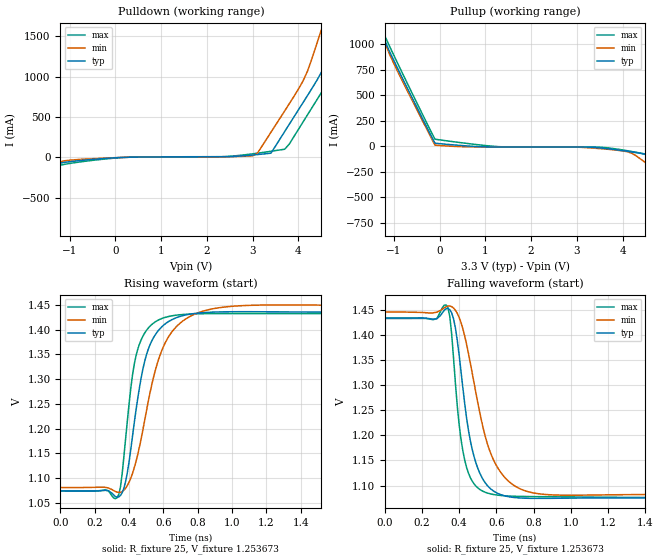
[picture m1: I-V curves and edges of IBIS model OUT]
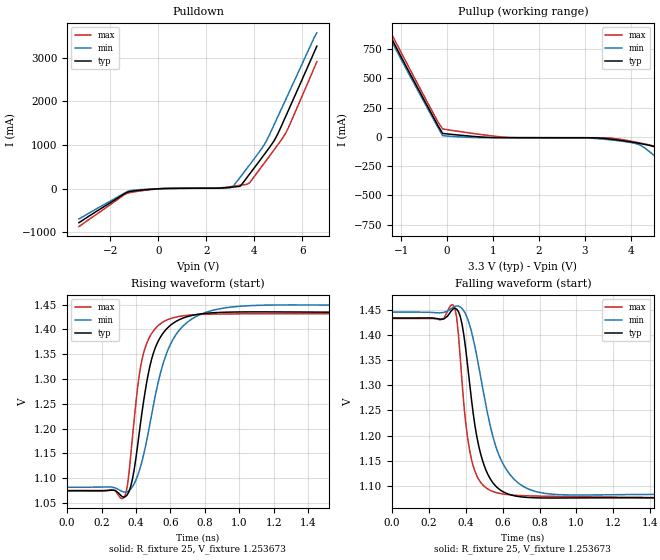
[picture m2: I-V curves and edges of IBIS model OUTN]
|   IBIS File of SG2520VHN C
|   LVDS, Vcc=3.3V, Io=7mA, fo<=212.5MHz
[IBIS Ver]   3.2
[File Name]   sg2520vhn_7m_33v.ibs
[File Rev]   1.0
[Date]   Sep. 23, 2020
[Source]
Fairchild Ensigna Lab's Method
[Notes]
Created by Minoru Kozaki
[Disclaimer]
Seiko Epson Corporation makes no warranty with respect to the
information contained herein.
[Copyright]
Copyright(C) 2020, Seiko Epson Corporation. All rights reserved.
|   Component
[Component]   SG2520VHN
[Manufacturer]  Seiko Epson Corporation
[Package]
R_pkg   17.7m   NA   NA
L_pkg   235p   NA   NA
C_pkg   208f   NA   NA
[Pin]   signal_name   model_name   R_pin   L_pin   C_pin
1   OE/ST   NC
2   NC   NC
3   GND   GND
4   OUT   OUT   17.7m   235p   208f
5   OUTN   OUTN   10.4m   129p   221f
6   VCC   POWER
[Diff Pin] inv_pin  vdiff  tdelay_typ
4   5   0   0
| Models and submodels in the file (2): OUT (Output), OUTN (Output)
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|   Model OUT
[Model]   OUT
Model_type   Output
Polarity   Non-Inverting
Vref = 1.25
Vmeas = 1.25
Rref = 25
Cref = 0
C_comp   4.5p   4.5p   4.5p
[Temperature Range]   25   105   -40
[Voltage Range]   3.3   2.97   3.63
[Pullup Reference]   3.3   2.97   3.63
[Pulldown Reference]   0   0   0
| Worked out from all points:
|   slope of the pulldown table from 0 to 0.495 V, typ, clamps not added: 59.9 ohm
|   slope of the pullup table from 0 to 0.495 V, typ, clamps not added: 26.2 ohm
|   falling waveform, R_fixture 25, V_fixture 1.253673: 20-80 % time 90.2ps typ, 136ps min, 64.6ps max; typ from 1.43 V to 1.07 V
|   rising waveform, R_fixture 25, V_fixture 1.253673: 20-80 % time 108ps typ, 155ps min, 80.6ps max; typ from 1.07 V to 1.43 V
[Pullup]
-3.3V     4.636A     4.476A     4.811A
-1.3V     1.176A     1.178A     1.203A
-1.1V     936.4mA    909.9mA    988.4mA
-1V       841.7mA    812mA      893.1mA
-100mV    29.84mA    10.72mA    69.05mA
1.3V      -6.914mA   -7.163mA   -4.423mA
2.9V      -7.381mA   -7.911mA   -7.373mA
3.7V      -25.8mA    -30.57mA   -17.11mA
4.2V      -56.22mA   -67.88mA   -51.54mA
4.5V      -80.52mA   -160.5mA   -76.54mA
5V        -246mA     -323.5mA   -147.5mA
6.6V      -827.3mA   -836.8mA   -804.6mA
[Pulldown]
-3.3V     -809.5mA   -716.5mA   -913.3mA
-1.2V     -69.13mA   -51.35mA   -94.89mA
200mV     1.302mA    1.212mA    553uA
3V        30.18mA    20.64mA    44.91mA
3.4V      52.94mA    312.2mA    76.77mA
3.8V      410.9mA    665.3mA    164.9mA
4.2V      768.6mA    1.072A     529.3mA
4.5V      1.053A     1.579A     801.7mA
4.8V      1.538A     2.102A     1.078A
4.9V      1.721A     2.277A     1.18A
5.2V      2.272A     2.804A     1.692A
6.6V      4.638A     5.026A     4.23A
[Falling Waveform]
R_fixture = 25
V_fixture = 1.253673
V_fixture_min = 1.263010
V_fixture_max = 1.253579
0s        1.434V     1.445V     1.433V
340ps     1.453V     1.457V     1.454V
360ps     1.444V     1.456V     1.401V
380ps     1.414V     1.449V     1.304V
430ps     1.263V     1.398V     1.151V
490ps     1.145V     1.284V     1.099V
570ps     1.093V     1.164V     1.083V
690ps     1.076V     1.101V     1.079V
880ps     1.074V     1.082V     1.078V
4ns       1.074V     1.081V     1.074V
[Rising Waveform]
R_fixture = 25
V_fixture = 1.253673
V_fixture_min = 1.263010
V_fixture_max = 1.253579
0s        1.074V     1.081V     1.074V
330ps     1.061V     1.072V     1.06V
350ps     1.065V     1.071V     1.082V
380ps     1.093V     1.08V      1.18V
450ps     1.26V      1.147V     1.36V
520ps     1.368V     1.269V     1.406V
620ps     1.414V     1.38V      1.426V
770ps     1.432V     1.429V     1.432V
1.05ns    1.436V     1.448V     1.433V
4ns       1.434V     1.446V     1.433V
[Ramp]
R_load = 25
dV/dt_r   0.21607/108.06p   0.21845/154.31p   0.21539/80.82p
dV/dt_f   0.21607/90.19p   0.21845/135.99p   0.21539/64.39p
|   Model OUTN
[Model]   OUTN
Model_type   Output
Polarity   Inverting
Vref = 1.25
Vmeas = 1.25
Rref = 25
Cref = 0
C_comp   4.5p   4.5p   4.5p
[Temperature Range]   25   105   -40
[Voltage Range]   3.3   2.97   3.63
[Pullup Reference]   3.3   2.97   3.63
[Pulldown Reference]   0   0   0
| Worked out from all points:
|   slope of the pulldown table from 0 to 0.495 V, typ, clamps not added: 60.3 ohm
|   slope of the pullup table from 0 to 0.495 V, typ, clamps not added: 26.4 ohm
|   falling waveform, R_fixture 25, V_fixture 1.253673: 20-80 % time 91.8ps typ, 136ps min, 66.7ps max; typ from 1.43 V to 1.07 V
|   rising waveform, R_fixture 25, V_fixture 1.253673: 20-80 % time 109ps typ, 155ps min, 81.7ps max; typ from 1.07 V to 1.43 V
[Pullup]
-3.3V     3.261A     3.196A     3.332A
-1.4V     986.7mA    967.8mA    1.027A
-1.3V     908.9mA    886mA      949.5mA
-1.2V     832.8mA    809.4mA    872.4mA
-200mV    95.43mA    80.01mA    126.2mA
-100mV    29.59mA    10.68mA    67.95mA
1.3V      -6.914mA   -7.163mA   -4.437mA
3.4V      -12.72mA   -19.72mA   -7.667mA
4.1V      -49.54mA   -56.22mA   -44.02mA
4.5V      -82.16mA   -156.7mA   -77.26mA
5V        -237.1mA   -311.1mA   -141.2mA
6.6V      -798.3mA   -812.4mA   -762.7mA
[Pulldown]
-3.3V     -781.1mA   -696.2mA   -870.7mA
-1.3V     -85.52mA   -71.69mA   -107.6mA
100mV     -968uA     -558uA     -2.96mA
2.4V      9.232mA    8.771mA    11.14mA
3.1V      35.22mA    39.1mA     51.92mA
3.4V      52.41mA    254.7mA    75.79mA
3.8V      333.6mA    543.2mA    132.1mA
4.5V      847.8mA    1.094A     649.1mA
4.9V      1.174A     1.558A     948.8mA
5.2V      1.528A     1.916A     1.179A
5.4V      1.775A     2.155A     1.378A
6.6V      3.265A     3.571A     2.909A
[Falling Waveform]
R_fixture = 25
V_fixture = 1.253673
V_fixture_min = 1.263010
V_fixture_max = 1.253579
0s        1.434V     1.445V     1.433V
340ps     1.453V     1.457V     1.454V
360ps     1.446V     1.457V     1.401V
380ps     1.421V     1.452V     1.305V
430ps     1.274V     1.408V     1.154V
490ps     1.151V     1.298V     1.103V
570ps     1.097V     1.171V     1.086V
690ps     1.079V     1.104V     1.081V
880ps     1.076V     1.083V     1.079V
4ns       1.074V     1.082V     1.075V
[Rising Waveform]
R_fixture = 25
V_fixture = 1.253673
V_fixture_min = 1.263010
V_fixture_max = 1.253579
0s        1.074V     1.082V     1.075V
330ps     1.062V     1.072V     1.06V
350ps     1.066V     1.072V     1.084V
380ps     1.098V     1.083V     1.183V
420ps     1.193V     1.116V     1.31V
450ps     1.267V     1.155V     1.359V
510ps     1.361V     1.262V     1.401V
620ps     1.413V     1.383V     1.424V
1.05ns    1.435V     1.448V     1.432V
4ns       1.434V     1.446V     1.432V
[Ramp]
R_load = 25
dV/dt_r   0.21405/107.32p   0.21633/152.25p   0.21338/80.84p
dV/dt_f   0.21405/90.92p   0.21633/134.96p   0.21338/65.97p
